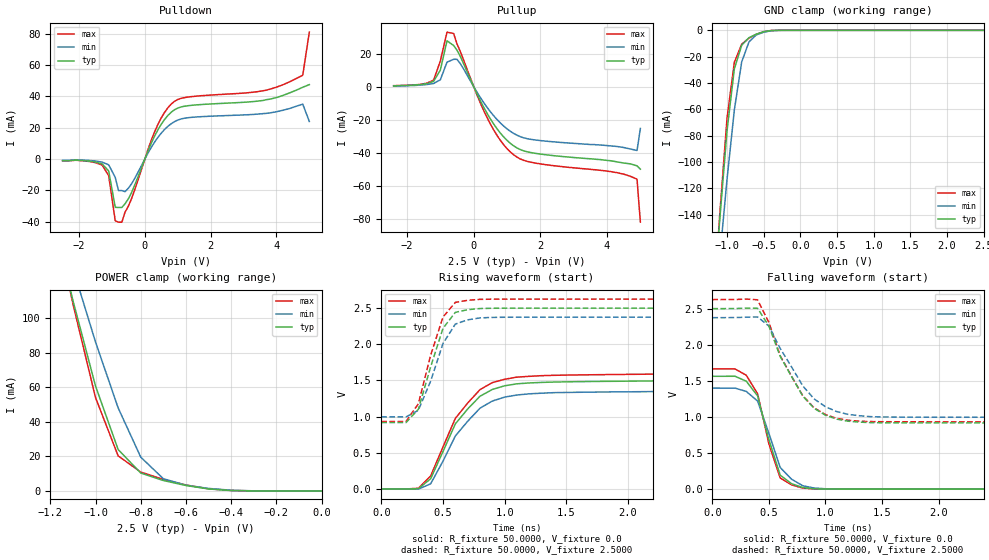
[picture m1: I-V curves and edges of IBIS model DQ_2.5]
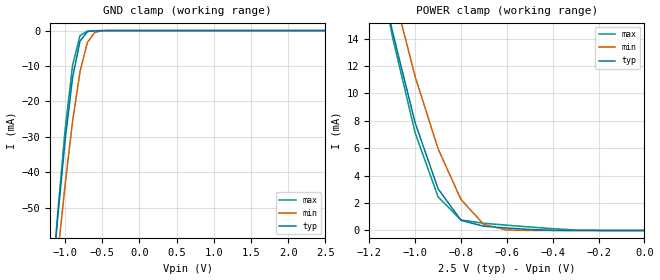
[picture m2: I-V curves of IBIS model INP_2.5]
|*** ISSI Synchronous Sram IBIS Model ***
[IBIS ver]	3.2
[File name]	is61vf12832165bga.ibs
[File Rev]	1.0
[Date]	May 13,2013
[Notes]
|--- Version History --------------------------------
|1.0: prelimiary
[Disclaimer]	This information is for modeling purpose only
		and is not guaranteed
[Copyright]	INTEGRATED SILICON SOLUTION, INC. 2011
[Component]	IS61VF12832_165BGA
[Manufacturer]	ISSI
[Package]
| variable   typ   min   max
R_pkg		100.34m			23.84m			218.59m
L_pkg		1.3400nH		0.3700nH		3.0300nH
C_pkg		41.410pF		0.4200pF		150.38pF
[Pin]  signal_name   model_name   R_pin   L_pin   C_pin
R11   A   INP_2.5
R10   A   INP_2.5
R9   A   INP_2.5
R8   A   INP_2.5
R7   TCK   INP_2.5
R6   A0   INP_2.5
R5   TMS   INP_2.5
R4   A   INP_2.5
R3   A   INP_2.5
R2   NC   NC
R1   MODE   INP_2.5
P11   NC   NC
P10   A   INP_2.5
P9   A   INP_2.5
P8   A   INP_2.5
P7   TDO   DQ_2.5
P6   A1   INP_2.5
P5   TDI   INP_2.5
P4   A   INP_2.5
P3   A   INP_2.5
P2   NC   NC
P1   NC   NC
N11   DQPa   DQ_2.5
N10   NC   NC
N9   VDDQ   POWER
N8   VSS   GND
N7   NC   NC
N6   NC   NC
N5   NC   NC
N4   VSS   GND
N3   VDDQ   POWER
N2   NC   NC
N1   DQPd   DQ_2.5
M11   DQa   DQ_2.5
M10   DQa   DQ_2.5
M9   VDDQ   POWER
M8   VDD   POWER
M7   VSS   GND
M6   VSS   GND
M5   VSS   GND
M4   VDD   POWER
M3   VDDQ   POWER
M2   DQd   DQ_2.5
M1   DQd   DQ_2.5
L11   DQa   DQ_2.5
L10   DQa   DQ_2.5
L9   VDDQ   POWER
L8   VDD   POWER
L7   VSS   GND
L6   VSS   GND
L5   VSS   GND
L4   VDD   POWER
L3   VDDQ   POWER
L2   DQd   DQ_2.5
L1   DQd   DQ_2.5
K11   DQa   DQ_2.5
K10   DQa   DQ_2.5
K9   VDDQ   POWER
K8   VDD   POWER
K7   VSS   GND
K6   VSS   GND
K5   VSS   GND
K4   VDD   POWER
K3   VDDQ   POWER
K2   DQd   DQ_2.5
K1   DQd   DQ_2.5
J11   DQa   DQ_2.5
J10   DQa   DQ_2.5
J9   VDDQ   POWER
J8   VDD   POWER
J7   VSS   GND
J6   VSS   GND
J5   VSS   GND
J4   VDD   POWER
J3   VDDQ   POWER
J2   DQd   DQ_2.5
J1   DQd   DQ_2.5
H11   ZZ   INP_2.5
H10   NC   NC
H9   NC   NC
H8   VDD   POWER
H7   VSS   GND
H6   VSS   GND
H5   VSS   GND
H4   VDD   POWER
H3   NC   NC
H2   VSS   GND
H1   NC   NC
G11   DQb   DQ_2.5
G10   DQb   DQ_2.5
G9   VDDQ   POWER
G8   VDD   POWER
G7   VSS   GND
G6   VSS   GND
G5   VSS   GND
G4   VDD   POWER
G3   VDDQ   POWER
G2   DQc   DQ_2.5
G1   DQc   DQ_2.5
F11   DQb   DQ_2.5
F10   DQb   DQ_2.5
F9   VDDQ   POWER
F8   VDD   POWER
F7   VSS   GND
F6   VSS   GND
F5   VSS   GND
F4   VDD   POWER
F3   VDDQ   POWER
F2   DQc   DQ_2.5
F1   DQc   DQ_2.5
E11   DQb   DQ_2.5
E10   DQb   DQ_2.5
E9   VDDQ   POWER
E8   VDD   POWER
E7   VSS   GND
E6   VSS   GND
E5   VSS   GND
E4   VDD   POWER
E3   VDDQ   POWER
E2   DQc   DQ_2.5
E1   DQc   DQ_2.5
D11   DQb   DQ_2.5
D10   DQb   DQ_2.5
D9   VDDQ   POWER
D8   VDD   POWER
D7   VSS   GND
D6   VSS   GND
D5   VSS   GND
D4   VDD   POWER
D3   VDDQ   POWER
D2   DQc   DQ_2.5
D1   DQc   DQ_2.5
C11   DQPc   DQ_2.5
C10   NC   NC
C9   VDDQ   POWER
C8   VSS   GND
C7   VSS   GND
C6   VSS   GND
C5   VSS   GND
C4   VSS   GND
C3   VDDQ   POWER
C2   NC   NC
C1   DQPc   DQ_2.5
B11   NC   NC
B10   A   INP_2.5
B9   ADSPB   INP_2.5
B8   OEB   INP_2.5
B7   GWB   INP_2.5
B6   CLK   INP_2.5
B5   BWaB   INP_2.5
B4   BWdB   INP_2.5
B3   CE2   INP_2.5
B2   A   INP_2.5
B1   NC   NC
A11   NC   NC
A10   A   INP_2.5
A9   ADVB   INP_2.5
A8   ADSCB   INP_2.5
A7   BWEB   INP_2.5
A6   CE2B   INP_2.5
A5   BWbB   INP_2.5
A4   BWcB   INP_2.5
A3   CEB   INP_2.5
A2   A   INP_2.5
A1   NC   NC
| Models and submodels in the file (2): DQ_2.5 (3-state), INP_2.5 (Input)
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|   Model DQ_2.5
[Model]		DQ_2.5
Model_type	3-state
Polarity   Non-Inverting
Enable   Active-Low
Vmeas = 	0.7500V
Cref = 		5.0000pF
Rref = 		50.0000
Vref = 		1.2500V
C_comp   3.8290pF   3.3420pF   4.0300pF|
[Temperature Range]	  25.0000   100.0000   0.0
[Voltage Range]   2.5000V   2.3750V   2.6250V
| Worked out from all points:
|   slope of the pulldown table from 0 to 0.375 V, typ, clamps not added: 21.1 ohm
|   slope of the pullup table from 0 to 0.375 V, typ, clamps not added: 24.7 ohm
|   GND clamp passes 1 mA (typ) near -0.49 V on its own axis
|   POWER clamp passes 1 mA (typ) near -0.48 V on its own axis
|   rising waveform, R_fixture 50.0000, V_fixture 0.0: 20-80 % time 314ps typ, 320ps min, 316ps max; typ from 0 V to 1.51 V
|   rising waveform, R_fixture 50.0000, V_fixture 2.5000: 20-80 % time 170ps typ, 187ps min, 169ps max; typ from 0.918 V to 2.5 V
|   falling waveform, R_fixture 50.0000, V_fixture 0.0: 20-80 % time 169ps typ, 190ps min, 167ps max; typ from 1.56 V to 0 V
|   falling waveform, R_fixture 50.0000, V_fixture 2.5000: 20-80 % time 314ps typ, 336ps min, 308ps max; typ from 2.5 V to 0.918 V
[Pulldown]
|Voltage	  I(typ)   I(min)   I(max)
-2.5V     -1mA       -900uA     -1.1mA
-1.3V     -3.1mA     -1.98mA    -3.85mA
-1.1V     -7.6mA     -3.69mA    -10.56mA
-900mV    -30.82mA   -11.68mA   -39.46mA
-800mV    -30.93mA   -20.13mA   -40.31mA
-700mV    -30.93mA   -20.13mA   -40.31mA
-400mV    -21.21mA   -15.69mA   -25.04mA
300mV     14.77mA    10.9mA     17.5mA
800mV     29.84mA    22.52mA    35.05mA
3.7V      37.9mA     29.16mA    43.99mA
4.8V      45.8mA     35.01mA    53.46mA
5V        47.5mA     23.97mA    81.01mA
[Pullup]
|Voltage	  I(typ)   I(min)   I(max)
-2.4V     400uA      360uA      550uA
-1.2V     3.2mA      1.89mA     3.96mA
-1V       9.97mA     4.104mA    15.48mA
-800mV    27.74mA    14.77mA    33.01mA
-600mV    24.84mA    16.54mA    32.14mA
-400mV    18.24mA    13.88mA    21.25mA
300mV     -12.46mA   -9.666mA   -14.47mA
1V        -32.57mA   -25.6mA    -37.58mA
1.6V      -39.48mA   -31.55mA   -45.26mA
4.1V      -44.9mA    -35.91mA   -51.48mA
4.9V      -48mA      -38.7mA    -56.1mA
5V        -50mA      -25.39mA   -82.14mA
[GND_clamp]
|Voltage	  I(typ)   I(min)   I(max)
-2.5V     -1.238A    -1.081A    -1.377A
-1.2V     -220.2mA   -237.3mA   -225.5mA
-1.1V     -144.4mA   -173.5mA   -140.5mA
-1V       -76.37mA   -113.2mA   -66.76mA
-900mV    -29.2mA    -60.35mA   -24.24mA
-800mV    -11.34mA   -23.99mA   -10.52mA
-700mV    -5.573mA   -8.7mA     -5.892mA
-600mV    -2.907mA   -3.457mA   -3.011mA
-500mV    -1.075mA   -1.408mA   -999.8uA
-300mV    -9.492uA   -41.34uA   -5.052uA
2.5V      40.97nA    416.1nA    43nA
[POWER_clamp]
|Voltage	  I(typ)   I(min)   I(max)
-2.5V     946.2mA    803.1mA    1.061A
-1.2V     165.2mA    174.2mA    170.3mA
-1.1V     110.4mA    129mA      108.4mA
-1V       60.76mA    86.26mA    54.07mA
-900mV    23.99mA    48.12mA    20.31mA
-800mV    10.36mA    19.57mA    10.92mA
-700mV    6.025mA    7.051mA    6.647mA
-600mV    3.142mA    3.321mA    3.423mA
-500mV    1.147mA    1.448mA    1.242mA
-400mV    194.4uA    400.6uA    266.4uA
0V        40.97nA    40.9nA     75.05nA
[Ramp]
| variable   typ   min   max
dV/dt_r		0.9042/0.2795n   0.7824/0.2922n   0.9954/0.2697n
dV/dt_f		0.9493/0.2827n   0.8275/0.2702n   1.0156/0.3061n
R_load =	50.0000
[Rising Waveform]
R_fixture=	50.0000
V_fixture=	0.0
V_fixture_min=	0.0
V_fixture_max=	0.0
|time   V(typ)   V(min)   V(max)
0s        0V         0V         0V
300ps     3.703mV    -2.782mV   10.28mV
400ps     140.9mV    71.68mV    179.8mV
600ps     899.4mV    732.5mV    975.4mV
800ps     1.282V     1.117V     1.373V
900ps     1.375V     1.216V     1.47V
1ns       1.427V     1.27V      1.516V
1.2ns     1.466V     1.315V     1.557V
1.6ns     1.484V     1.337V     1.577V
5ns       1.507V     1.359V     1.602V
[Rising Waveform]
R_fixture=	50.0000
V_fixture=	2.5000
V_fixture_min=	2.3750
V_fixture_max=	2.6250
|time   V(typ)   V(min)   V(max)
0s        917.8mV    995.8mV    932.4mV
200ps     917.8mV    995.8mV    932.6mV
300ps     1.101V     1.087V     1.177V
400ps     1.689V     1.492V     1.849V
500ps     2.221V     2.011V     2.377V
600ps     2.441V     2.279V     2.579V
700ps     2.478V     2.338V     2.608V
800ps     2.494V     2.365V     2.621V
900ps     2.498V     2.372V     2.623V
5ns       2.5V       2.375V     2.625V
[Falling Waveform]
R_fixture=	50.0000
V_fixture=	0.0
V_fixture_min=	0.0
V_fixture_max=	0.0
|time   V(typ)   V(min)   V(max)
0s        1.563V     1.4V       1.665V
200ps     1.563V     1.399V     1.665V
300ps     1.495V     1.353V     1.577V
400ps     1.292V     1.22V      1.321V
500ps     684mV      773.4mV    627.2mV
600ps     194.2mV    300.3mV    154.3mV
700ps     76.23mV    138.2mV    59.74mV
800ps     22.14mV    46.86mV    14.45mV
1.1ns     594.5uV    1.764mV    405.6uV
5ns       23.76uV    34.03uV    20.31uV
[Falling Waveform]
R_fixture=	50.0000
V_fixture=	2.5000
V_fixture_min=	2.3750
V_fixture_max=	2.6250
|time   V(typ)   V(min)   V(max)
0s        2.5V       2.375V     2.625V
400ps     2.505V     2.385V     2.622V
500ps     2.259V     2.258V     2.31V
600ps     1.839V     1.948V     1.847V
800ps     1.289V     1.429V     1.292V
900ps     1.119V     1.25V      1.126V
1ns       1.024V     1.142V     1.033V
1.1ns     969.7mV    1.075V     979.6mV
1.5ns     919.4mV    999.8mV    933.8mV
5ns       917.8mV    995.8mV    932.4mV
|   Model INP_2.5
[Model]		INP_2.5
Model_type	Input
Polarity   Non-Inverting
Enable   Active-Low
Vinl = 		0.8000V
Vinh = 		2.0000V
C_comp   3.8290pF   3.3420pF   4.0300pF|
[Temperature Range]	  25.0000   100.0000   0.0
[Voltage Range]   2.5000V   2.3750V   2.6250V
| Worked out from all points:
|   GND clamp passes 1 mA (typ) near -0.73 V on its own axis
|   POWER clamp passes 1 mA (typ) near -0.81 V on its own axis
[GND_clamp]
|Voltage	  I(typ)   I(min)   I(max)
-2.5V     -434.7mA   -399mA     -475.2mA
-1.2V     -76.89mA   -84.89mA   -78.19mA
-1.1V     -52.83mA   -63.46mA   -51.66mA
-1V       -30.98mA   -43.42mA   -27.92mA
-900mV    -13.28mA   -25.61mA   -9.811mA
-800mV    -2.971mA   -11.61mA   -1.401mA
-700mV    -287uA     -3.303mA   -148.3uA
-600mV    -52.18uA   -480.7uA   -48.72uA
-500mV    -11.21uA   -45.78uA   -9.079uA
2.5V      40.19nA    40.4nA     42.61nA
[POWER_clamp]
|Voltage	  I(typ)   I(min)   I(max)
-2.5V     189.7mA    171.9mA    207.8mA
-1.2V     22.77mA    25.28mA    23.03mA
-1.1V     14.57mA    17.73mA    14.18mA
-1V       7.84mA     11.21mA    7.108mA
-900mV    3.038mA    5.954mA    2.453mA
-800mV    736uA      2.255mA    762.7uA
-700mV    308.2uA    432.8uA    524.6uA
-600mV    181.1uA    36.29uA    386.3uA
-400mV    10.09uA    187.6nA    130.9uA
-300mV    415nA      89.24nA    33.9uA
0V        40.19nA    23.22nA    74.57nA
